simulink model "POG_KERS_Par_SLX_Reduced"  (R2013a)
settings: Solver=ode45  StartTime=0.0  StopTime=10.0  RelTol=1e-3
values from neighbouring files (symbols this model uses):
  bth = b_1+b_2*R2^2+b_b*Rbth.^2+b_3*R3th.^2    [POG_KERS_Par_SLX_m.m]
  dJ_dth = eval(dJ_dth)    [POG_KERS_Par_SLX_m.m]
  Jth = J_1+J_2*R2^2+J_b*Rbth.^2+J_3*R3th.^2    [POG_KERS_Par_SLX_m.m]
  R3th = r_1*r2th./(r_2.*r3th)    [POG_KERS_Par_SLX_m.m]
  Rbth = r_1*r2th./(r_2.*r_b)    [POG_KERS_Par_SLX_m.m]
  T_1_0 = 0*Nm    [POG_KERS_Par_SLX_m.m]    (also in POG_KERS_SLX_m.m = 0)
  T_3_0 = 0*Nm    [POG_KERS_Par_SLX_m.m]
  Tc = Ts    (= 0.0015)    [POG_KERS_Par_SLX_m.m]
  th_0 = th(1)    [POG_KERS_Par_SLX_m.m]
  Th_in = th    [POG_KERS_Par_SLX_m.m]
  Ts = Tfin/Nr_Ts_Points    (= 0.0015)    [POG_KERS_Par_SLX_m.m]    (also in POG_KERS_SLX_m.m = 0.005)
  w_1_0 = 2000*rpm    [POG_KERS_Par_SLX_m.m]

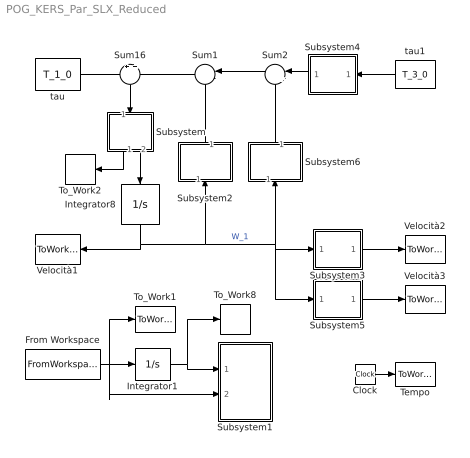
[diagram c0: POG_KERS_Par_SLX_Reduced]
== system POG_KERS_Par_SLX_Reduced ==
  Clock : Clock
  From Workspace : FromWorkspace  VariableName=[tt dot_th]  SampleTime=0
  Integrator1 : Integrator  InitialCondition=th_0  LowerSaturationLimit=0
  Integrator8 : Integrator  InitialCondition=w_1_0  LowerSaturationLimit=0
  Subsystem : Subsystem
  Subsystem1 : Subsystem
  Subsystem2 : Subsystem
  Subsystem3 : Subsystem
  Subsystem4 : Subsystem
  Subsystem5 : Subsystem
  Subsystem6 : Subsystem
  Sum1 : Sum  Inputs=|--
  Sum16 : Sum  Inputs=+|+
  Sum2 : Sum  Inputs=|++
  Tempo : ToWorkspace  VariableName=t  SampleTime=Tc
  To_Work1 : ToWorkspace  VariableName=dot_Th  SampleTime=Ts
  To_Work2 : ToWorkspace  VariableName=Jth_t  SampleTime=Ts
  To_Work8 : ToWorkspace  VariableName=Th  SampleTime=Ts
  Velocità1 : ToWorkspace  VariableName=w_1  SampleTime=Tc
  Velocità2 : ToWorkspace  VariableName=w_3  SampleTime=Tc
  Velocità3 : ToWorkspace  VariableName=w_b  SampleTime=Tc
  tau : Constant  Value=T_1_0
  tau1 : Constant  Value=T_3_0
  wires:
  Clock/1 -> Tempo/1
  Integrator8/1 -> Velocità1/1, Subsystem2/1(w_1), Subsystem5/1(In), Subsystem6/1(w_1), Subsystem3/1(In)  "W_1"
  Sum1/1 -> Sum16/2
  Subsystem2/1(Nth) -> Sum1/2
  tau/1 -> Sum16/1
  Subsystem6/1(b_th) -> Sum2/2
  Sum2/1 -> Sum1/1
  Subsystem4/1(Out) -> Sum2/1
  Subsystem3/1(Out) -> Velocità2/1
  tau1/1 -> Subsystem4/1(In)
  Sum16/1 -> Subsystem/1(In1)
  Subsystem/2(Out1) -> Integrator8/1
  From Workspace/1 -> Subsystem1/2(dot_th), To_Work1/1, Integrator1/1
  Integrator1/1 -> To_Work8/1, Subsystem1/1(th)
  Subsystem5/1(Out) -> Velocità3/1
  Subsystem/1(Jth) -> To_Work2/1

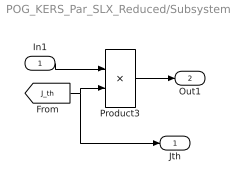
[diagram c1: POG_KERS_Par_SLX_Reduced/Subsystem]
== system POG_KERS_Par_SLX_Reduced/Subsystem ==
  In1 : Inport
  Product3 : Product  Inputs=*/
  Jth : Outport
  Out1 : Outport  Port=2
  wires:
  In1/1 -> Product3/1
  Product3/1 -> Out1/1
  [J_th] -> Jth/1, Product3/2

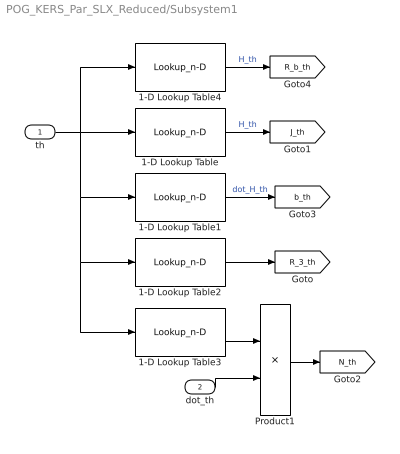
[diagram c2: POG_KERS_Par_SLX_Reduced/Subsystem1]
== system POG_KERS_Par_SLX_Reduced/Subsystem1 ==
  th : Inport
  dot_th : Inport  Port=2
  1-D Lookup Table : Lookup_n-D  NumberOfTableDimensions=1  BreakpointsForDimension1=Th_in  Table=Jth  RndMeth=Simplest
  1-D Lookup Table1 : Lookup_n-D  NumberOfTableDimensions=1  BreakpointsForDimension1=Th_in  Table=bth  RndMeth=Simplest
  1-D Lookup Table2 : Lookup_n-D  NumberOfTableDimensions=1  BreakpointsForDimension1=Th_in  Table=R3th  RndMeth=Simplest
  1-D Lookup Table3 : Lookup_n-D  NumberOfTableDimensions=1  BreakpointsForDimension1=Th_in  Table=dJ_dth  RndMeth=Simplest
  1-D Lookup Table4 : Lookup_n-D  NumberOfTableDimensions=1  BreakpointsForDimension1=Th_in  Table=Rbth  RndMeth=Simplest
  Product1 : Product
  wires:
  1-D Lookup Table/1 -> [J_th]  "H_th"
  1-D Lookup Table1/1 -> [b_th]  "dot_H_th"
  1-D Lookup Table2/1 -> [R_3_th]
  Product1/1 -> [N_th]
  1-D Lookup Table3/1 -> Product1/1
  dot_th/1 -> Product1/2
  1-D Lookup Table4/1 -> [R_b_th]  "H_th"
  th/1 -> 1-D Lookup Table4/1, 1-D Lookup Table1/1, 1-D Lookup Table2/1, 1-D Lookup Table3/1, 1-D Lookup Table/1

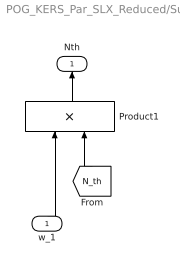
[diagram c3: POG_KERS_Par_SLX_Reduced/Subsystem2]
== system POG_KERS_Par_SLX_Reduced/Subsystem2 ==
  w_1 : Inport
  Product1 : Product
  Nth : Outport
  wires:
  w_1/1 -> Product1/1
  Product1/1 -> Nth/1
  [N_th] -> Product1/2

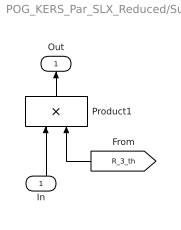
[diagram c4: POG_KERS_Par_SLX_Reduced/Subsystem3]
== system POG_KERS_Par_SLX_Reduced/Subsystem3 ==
  In : Inport
  Product1 : Product
  Out : Outport
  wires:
  Product1/1 -> Out/1
  In/1 -> Product1/1
  [R_3_th] -> Product1/2

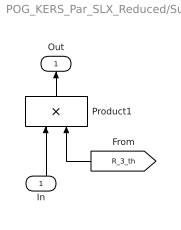
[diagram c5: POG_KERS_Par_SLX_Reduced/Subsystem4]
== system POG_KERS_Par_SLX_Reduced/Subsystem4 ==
  In : Inport
  Product1 : Product
  Out : Outport
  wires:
  [R_3_th] -> Product1/2
  In/1 -> Product1/1
  Product1/1 -> Out/1

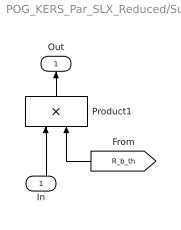
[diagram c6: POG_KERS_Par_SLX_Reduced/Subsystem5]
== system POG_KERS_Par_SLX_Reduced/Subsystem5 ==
  In : Inport
  Product1 : Product
  Out : Outport
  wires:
  [R_b_th] -> Product1/2
  In/1 -> Product1/1
  Product1/1 -> Out/1

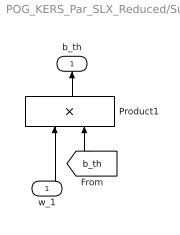
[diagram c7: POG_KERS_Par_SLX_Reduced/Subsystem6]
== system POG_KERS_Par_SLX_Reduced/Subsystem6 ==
  w_1 : Inport
  Product1 : Product
  b_th : Outport
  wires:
  [b_th] -> Product1/2
  Product1/1 -> b_th/1
  w_1/1 -> Product1/1
